{attribute 'qualified_only'}
{attribute 'strict'}
TYPE E_SboControlState :
(
	Unselected:=0,
	Select_PerformTest:=1,
	WaitForSelection:=2,
	Ready:=3,
	WaitForActivationTime:=4,
	PerformTest:=5,
	WaitForExecution:=6,
	MirrorBlockedCommand:=7,
	WaitForChange:=8,
	EndSelection:=9
);
END_TYPE
